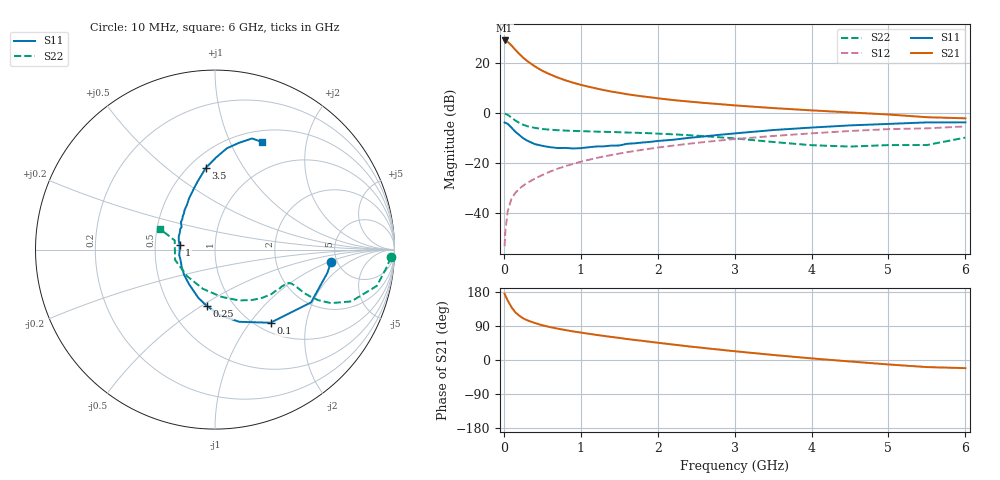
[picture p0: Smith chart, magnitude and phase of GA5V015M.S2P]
! Infineon Technologies  Discrete & RF Semiconductors
! BF775
! Si NPN RF Bipolar Junction Transistor in SOT23
! VCE = 5 V  IC = 15 mA
! Common Emitter S-Parameters:  May  1996
# GHz  S  MA  R  50
!  f  S11  S21  S12  S22
! GHz  MAG  ANG  MAG  ANG  MAG  ANG  MAG  ANG
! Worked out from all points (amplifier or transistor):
!   36 points, 10 MHz to 6 GHz, reference 50 ohm
!   highest |S21| = 29.0 dB at 10 MHz (marker M1)
!   |S21| within 3 dB of that: start of sweep to 128.2 MHz
!   unconditionally stable (mu >= 1): 474.6 MHz to 2.928 GHz
!   at 250 MHz: K = 0.78, MSG = 25.6 dB, |S12| = -29.0 dB
!   at 1.4 GHz: K = 1.10, MAG = 10.7 dB, |S12| = -16.7 dB
!   at 6 GHz: K = 0.93, MSG = 1.6 dB, |S12| = -5.3 dB
!   S11 on the Smith chart (normalised r, x): 10 MHz: 4.45, -1.06; 100 MHz: 1.15, -1.27; 250 MHz: 0.75, -0.52; 1 GHz: 0.67, +0.04; 3.5 GHz: 0.60, +0.70; 6 GHz: 0.63, +1.33
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0.01  0.65 -6.1  28.25 174.8  0.0022 91.6  0.9795 -2.5
0.02  0.6392 -11.8  28 170.0  0.0044 81.0  0.9662 -5.2
0.05  0.6107 -28.8  26.49 157.0  0.0109 78.5  0.9245 -12.6
0.1  0.5116 -52.8  22.34 139.2  0.0197 69.8  0.8127 -20.8
0.15  0.4241 -71.5  18.37 125.7  0.0256 65.7  0.7111 -24.8
0.2  0.3663 -85.9  15.28 117.0  0.0307 64.8  0.6395 -26.1
0.25  0.3164 -98.5  12.86 110.1  0.0355 64.5  0.5869 -26.2
0.3  0.284 -109.2  11.08 105.1  0.0399 65.7  0.5507 -25.9
0.4  0.2411 -126.8  8.641 97.8  0.0489 67.0  0.5074 -24.8
0.5  0.2222 -140.8  7.009 91.7  0.0579 67.7  0.4806 -24.2
0.6  0.209 -152.6  5.941 86.9  0.0678 68.6  0.4674 -24.0
0.7  0.2005 -163.0  5.14 82.7  0.0775 68.8  0.456 -24.2
0.8  0.2017 -171.1  4.521 79.0  0.0871 68.2  0.4476 -24.6
1  0.1995 172.2  3.677 72.4  0.1067 67.8  0.4363 -26.2
1.1  0.2079 165.9  3.373 69.4  0.1163 67.4  0.4317 -27.5
1.3  0.217 155.1  2.883 63.6  0.1361 65.8  0.4228 -29.8
1.6  0.2438 141.2  2.386 55.4  0.1654 63.4  0.4093 -34.2
2.2  0.2938 122.2  1.822 40.8  0.2243 57.6  0.3773 -45.2
3.5  0.459 96.3  1.261 13.3  0.3491 42.2  0.2649 -82.5
4.5  0.5683 83.3  1.031 -3.9  0.4395 29.2  0.2147 -136.7
5.5  0.6525 71.6  0.828 -18.7  0.4962 14.3  0.2304 167.1
6  0.6543 66.4  0.787 -21.5  0.5425 10.1  0.3247 159.6
